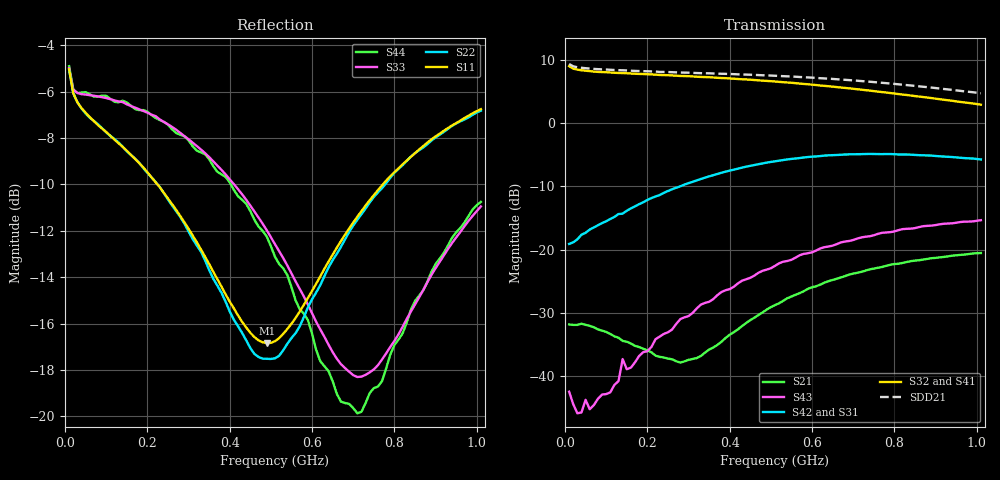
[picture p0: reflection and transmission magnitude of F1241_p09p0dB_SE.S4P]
! Integrated Device Technology
! Corporate Headquarters
! 6024 Silver Creek Valley Road
! San Jose, CA 95138  USA
! Phone:  1-408-284-8200
! Toll Free:  1-800-223-1366
! Webpage:  http://www.idt.com/
! Timing and RF Division
! 515 Groton Road, Suite 102
! Westford, MA 01886-6024
! Device:  F1241
! Description: Dual Intermediate Frequency Digital Variable Gain Amplifier
! Frequency:  10.0 -  500.00 MHz
! Package:  5x5 mm QFN Plastic Package: 32 pin
! Ports:  8 RF, 20 DC
!  Pin  1  = GA3  Pin 17  = RF OUT_B+
!  Pin  2  = GA4  Pin 18  = RF OUT_B-
!  Pin  3  = GA5  Pin 19  = STBY_B
!  Pin  4  = ISET_A  Pin 20  = Ground
!  Pin  5  = ISET_B  Pin 21  = Ground
!  Pin  6  = GB5  Pin 22  = STB_A
!  Pin  7  = GB4  Pin 23  = RF OUT_A-  = Port 4
!  Pin  8  = GB3  Pin 24  = RF OUT_A+  = Port 3
!  Pin  9  = GB2  Pin 25  = NO CONNECT
!  Pin 10  = GB1  Pin 26  = NO CONNECT
!  Pin 11  = RF IN_B+  Pin 27  = VCC
!  Pin 12  = RF IN_B-  Pin 28  = Ground
!  Pin 13  = Ground  Pin 29  = RF IN_A-  = Port 2
!  Pin 14  = VCC  Pin 30  = RF IN_A+  = Port 1
!  Pin 15  = NO CONNECT  Pin 31  = GA1
!  Pin 16  = NO CONNECT  Pin 32  = GA2
! State:  11
! Gain State:  9.0 dB
! Voltages:  Vcc = +5.00 Volts  Icc approximately 160.0 mA or 80 mA per channel.
! Data:  The device was measured on a custom evaluation board which has
!  individual transmission lines to the RF pins.  Data was collected
!  using a calibrated network analyzer.  The evaluation board was
!  de-embedded using a port reference technique.
!  The reference plane is the edge of the package pin.
!  Only Channel A was measured.
!  This data is in single-ended operation.  If your needs are balanced
!  or differential S-parameters then this file needs to be used a
!  linear simulator.
! Misc:  Lot Code  160028MY
!  Action Tracker AT004
! Date Measured:  2014-08-14
! Date:  2014-08-28  MJV
! Note:
!  Integrated Device Technology supplies this data as a sample of measured
!  data at the package pin for this product.  Your particular data for this
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# Hz S dB R 50
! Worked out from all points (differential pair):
!   101 points, 10 MHz to 1.01 GHz, reference 50 ohm
!   strongest paths, dB at 10 MHz, 260 MHz, 510 MHz, 760 MHz, 1.01 GHz:
!     S32: 9.1, 7.6, 6.6, 5.0, 3.0
!     S41: 9.1, 7.6, 6.5, 4.9, 2.8
!     S42: -19.1, -10.4, -6.0, -4.9, -5.7
!     S31: -19.1, -10.4, -6.1, -4.9, -5.8
!     S43: -42.5, -32.7, -22.6, -17.5, -15.3
!     S21: -31.8, -37.4, -28.8, -22.9, -20.5
!   taken as a pair (ports 2,1 in; 3,4 out), SDD21 dB: 9.4, 8.1, 7.5, 6.5, 4.8
!   lowest |S11| = -16.8 dB at 490 MHz (marker M1), VSWR 1.34, Z = 40 - j8.33 ohm
!   |S11| at or under -10 dB: 224.5 MHz to 771.9 MHz (547.4 MHz wide, 110 % of centre)
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1e7  -5.04 -20.3  -31.89 -1.0  -54.94 54.3  -17.90 13.7
     -31.85 -1.0  -5.05 -20.0  -17.92 13.3  -54.61 51.9
     -19.12 6.2  9.05 179.0  -4.99 -18.5  -42.66 147.8
     9.08 179.2  -19.09 6.1  -42.50 149.3  -4.90 -18.6
4e7  -6.71 -16.8  -31.78 -2.5  -47.19 65.3  -17.92 -0.7
     -31.73 -2.7  -6.72 -16.5  -17.90 -0.4  -47.59 65.4
     -17.61 19.4  8.41 172.1  -6.11 -8.5  -46.99 160.8
     8.43 171.9  -17.63 19.0  -45.78 155.7  -6.04 -8.0
1.4e8  -8.38 -31.0  -34.51 -4.8  -37.33 65.8  -18.23 -8.1
       -34.46 -6.8  -8.37 -29.7  -18.19 -7.9  -37.36 65.8
       -14.30 26.8  7.97 157.8  -6.45 -15.5  -38.38 136.9
       7.96 157.2  -14.30 26.3  -37.32 132.3  -6.39 -14.7
2.8e8  -11.36 -56.8  -36.43 32.9  -32.00 53.4  -18.03 -14.4
       -37.87 28.6  -11.40 -54.0  -18.00 -14.2  -32.00 52.7
       -10.00 22.6  7.50 138.9  -7.78 -29.5  -32.33 130.1
       7.48 138.2  -9.97 22.0  -30.99 127.0  -7.86 -27.7
4.9e8  -16.84 -134.9  -29.01 66.6  -27.95 33.6  -17.45 -28.0
       -29.49 72.6  -17.52 -133.8  -17.33 -28.0  -27.93 31.4
       -6.29 -2.7  6.72 110.8  -11.97 -57.5  -23.95 108.2
       6.64 110.0  -6.22 -4.3  -23.16 103.3  -12.25 -55.3
7.1e8  -11.39 148.0  -23.65 54.0  -25.82 13.6  -17.46 -46.2
       -23.66 58.7  -11.52 146.4  -17.17 -46.2  -25.80 10.2
       -4.95 -34.9  5.40 82.6  -18.30 -131.1  -18.97 78.8
       5.27 81.8  -4.89 -37.2  -18.24 75.9  -19.87 -138.0
1.01e9  -6.75 116.4  -20.87 32.0  -24.31 -10.7  -18.55 -69.1
        -20.54 34.6  -6.82 115.7  -18.06 -69.7  -24.34 -15.2
        -5.82 -73.0  2.95 49.2  -10.95 147.0  -15.97 42.5
        2.78 48.5  -5.72 -76.3  -15.34 40.0  -10.75 141.6
